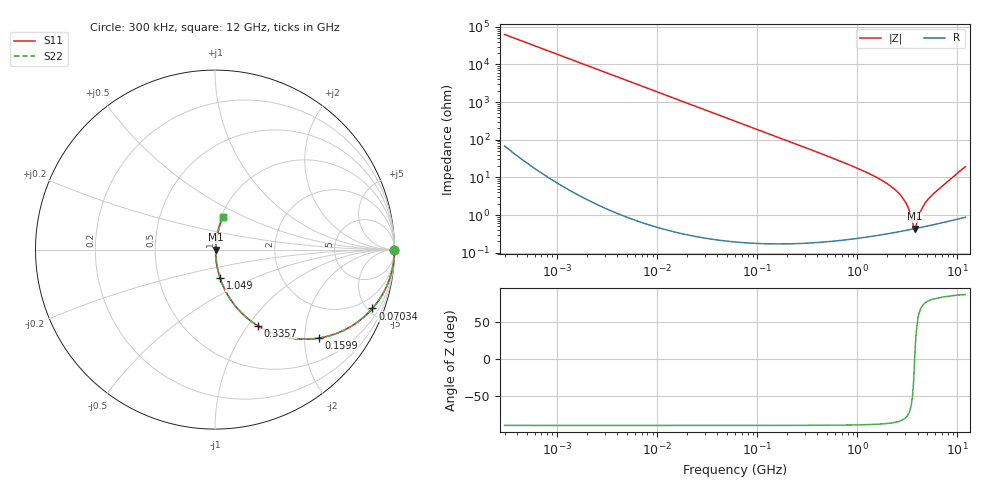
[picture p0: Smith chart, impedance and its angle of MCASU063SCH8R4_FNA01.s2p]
! MCASU063SCH8R4_FNA01  S-PARAMETER MODEL  ( General Type )
! Model Generated by TAIYO YUDEN Corporation (http://www.ty-top.com)
! Version 1.0
! TAIYO YUDEN Control No. 130801
! Copyright(c) 2013 TAIYO YUDEN CO.,LTD. All Rights Reserved.
! Product Description (link to TY-COMPAS)
! https://ds.yuden.co.jp/TYCOMPAS/or/detail?pn=MCASU063SCH8R4DFNA01&u=M
! Products Name : Multilayer Ceramic Capacitors
! Characteristics :
!  Capacitance : 8.4 pF , Rated Voltage : 50V , TCC : CH / C0H
!  Case Size : 0.6 x 0.3 / 0.024 x 0.012 [mm/inch] , Thickness : 0.3 / 0.012 [mm/inch]
!  (Conditions: Temperature = 25 degC , DC Bias Current/Voltage = 0A / 0V)
! External Node Assignments :
!  1  o---| |---o  2
! GND o---------o GND
! Frequency Range : 0.3MHz  -  12000MHz  [ 401 STEP ]
# MHz S RI R 50
! Freq[MHz].  S11 Real  S11 Imag  S21 Real  S21 Imag  S12 Real  S12 Imag  S22 Real  S22 Imag
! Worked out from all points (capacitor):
!   401 points, 300 kHz to 12 GHz, reference 50 ohm
!   read as one part in series: C = 8.45 pF near 316.3 kHz
!   lowest |Z| = 434 mohm at 3.741 GHz (marker M1)
!   series resonance near 3.736 GHz, so ESL is about 210 pH
!   S11 on the Smith chart (normalised r, x): 300 kHz: open; 70.34 MHz: 1.00, -5.36; 159.9 MHz: 1.00, -2.35; 335.7 MHz: 1.00, -1.11; 1.049 GHz: 1.00, -0.33; 12 GHz: 1.02, +0.38
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0.3  1 -0.00159  4.26e-06 0.00159  4.26e-06 0.00159  1 -0.00159
1.769972  0.9999 -0.00939  9.09e-05 0.00939  9.09e-05 0.00939  0.9999 -0.00939
10.44266  0.9969 -0.0553  0.00308 0.0553  0.00308 0.0553  0.9969 -0.0553
27.10171  0.9797 -0.1409  0.0203 0.1409  0.0203 0.1409  0.9797 -0.1409
60  0.9077 -0.2891  0.0923 0.2891  0.0923 0.2891  0.9077 -0.2891
70.33673  0.8774 -0.3276  0.1226 0.3276  0.1226 0.3276  0.8774 -0.3276
104.6549  0.7637 -0.4243  0.2363 0.4243  0.2363 0.4243  0.7637 -0.4243
159.8975  0.5803 -0.4928  0.4197 0.4928  0.4197 0.4928  0.5803 -0.4928
335.7268  0.2373 -0.4238  0.7627 0.4238  0.7627 0.4238  0.2373 -0.4238
353.9943  0.2184 -0.4115  0.7816 0.4115  0.7816 0.4115  0.2184 -0.4115
570.2811  0.0958 -0.2912  0.9042 0.2912  0.9042 0.2912  0.0958 -0.2912
1048.836  0.0289 -0.1603  0.9711 0.1603  0.9711 0.1603  0.0289 -0.1603
2088.533  0.00702 -0.0614  0.993 0.0614  0.993 0.0614  0.00702 -0.0614
2514.07  0.00519 -0.0407  0.9948 0.0407  0.9948 0.0407  0.00519 -0.0407
2947.191  0.00439 -0.024  0.9956 0.024  0.9956 0.024  0.00439 -0.024
3276.641  0.0042 -0.0132  0.9958 0.0132  0.9958 0.0132  0.0042 -0.0132
3547.679  0.00422 -0.00525  0.9958 0.00525  0.9958 0.00525  0.00422 -0.00525
3740.715  0.00432 0.000146  0.9957 -0.000146  0.9957 -0.000146  0.00432 0.000146
3944.255  0.00446 0.00448  0.9955 -0.00448  0.9955 -0.00448  0.00446 0.00448
4502.883  0.00501 0.0154  0.995 -0.0154  0.995 -0.0154  0.00501 0.0154
5140.631  0.00584 0.0263  0.9942 -0.0263  0.9942 -0.0263  0.00584 0.0263
12000  0.0431 0.1816  0.9569 -0.1816  0.9569 -0.1816  0.0431 0.1816
